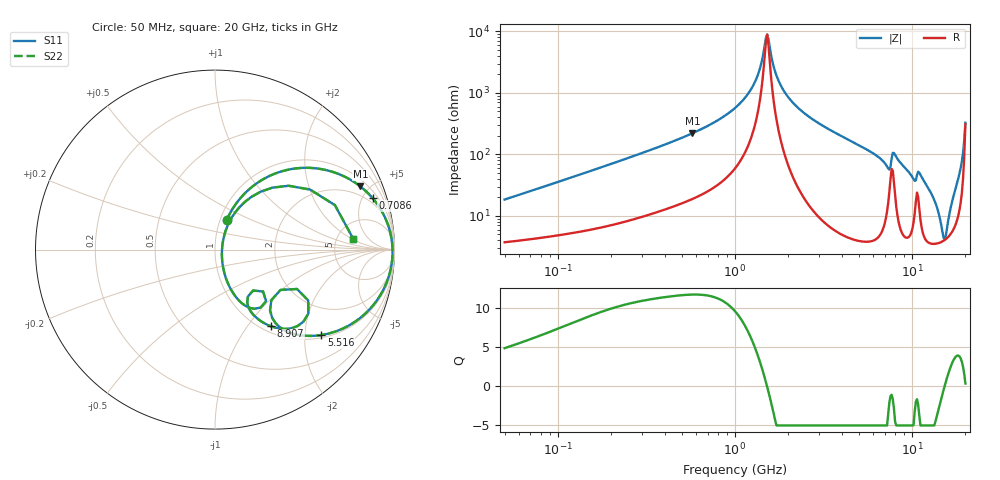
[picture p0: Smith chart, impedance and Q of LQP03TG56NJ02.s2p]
!Murata Part Number: LQP03TG56NJ02
!These Parameters are Measured in Series Mode Connection
!  o--[Z]--o
!Port1  Port2
!  o-------o
!Freq. Start=50[MHz] Stop=20[GHz], 401[Steps]
# Hz S RI R 50
!Freq.(Hz) S11(Real) S11(Imag) S21(Real) S21(Imag) S12(Real) S12(Imag) S22(Real) S22(Imag)
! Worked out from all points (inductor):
!   401 points, 50 MHz to 20 GHz, reference 50 ohm
!   read as one part in series: L = 57 nH near 51.52 MHz
!   highest Q = 11.7 at 574.5 MHz (marker M1), where L = 61 nH
!   self-resonance near 1.498 GHz
!   S11 on the Smith chart (normalised r, x): 50 MHz: 1.07, +0.36; 708.6 MHz: 1.51, +5.89; 5.516 GHz: 1.08, -2.43; 8.907 GHz: 1.10, -1.30; 20 GHz: 7.21, +2.10
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5e7  0.0645 0.1632  0.9355 -0.1632  0.9355 -0.1632  0.0645 0.1632
1.364002e8  0.2147 0.3561  0.7853 -0.3561  0.7853 -0.3561  0.2147 0.3561
3.721004e8  0.6283 0.4408  0.3717 -0.4408  0.3717 -0.4408  0.6283 0.4408
5.745257e8  0.8101 0.3517  0.1899 -0.3517  0.1899 -0.3517  0.8101 0.3517
7.08568e8  0.8776 0.2872  0.1224 -0.2872  0.1224 -0.2872  0.8776 0.2872
1e9  0.9539 0.1638  0.0461 -0.1638  0.0461 -0.1638  0.9539 0.1638
1.289994e9  0.9826 0.0648  0.0174 -0.0648  0.0174 -0.0648  0.9826 0.0648
1.521052e9  0.989 -0.00121  0.011 0.00121  0.011 0.00121  0.989 -0.00121
1.689197e9  0.988 -0.0439  0.012 0.0439  0.012 0.0439  0.988 -0.0439
1.848039e9  0.9839 -0.0809  0.0161 0.0809  0.0161 0.0809  0.9839 -0.0809
2.728004e9  0.9272 -0.2435  0.0728 0.2435  0.0728 0.2435  0.9272 -0.2435
5.515528e9  0.5926 -0.4759  0.4074 0.4759  0.4074 0.4759  0.5926 -0.4759
6.802353e9  0.3962 -0.4539  0.6038 0.4539  0.6038 0.4539  0.3962 -0.4539
7.442007e9  0.3139 -0.2821  0.6861 0.2821  0.6861 0.2821  0.3139 -0.2821
7.901521e9  0.5205 -0.3558  0.4795 0.3558  0.4795 0.3558  0.5205 -0.3558
8.907419e9  0.312 -0.4274  0.688 0.4274  0.688 0.4274  0.312 -0.4274
1.220001e10  0.1102 -0.2557  0.8898 0.2557  0.8898 0.2557  0.1102 -0.2557
1.354865e10  0.0562 -0.1447  0.9438 0.1447  0.9438 0.1447  0.0562 -0.1447
1.527346e10  0.0391 0.000819  0.9609 -0.000819  0.9609 -0.000819  0.0391 0.000819
1.800918e10  0.1649 0.2644  0.8351 -0.2644  0.8351 -0.2644  0.1649 0.2644
1.912117e10  0.4103 0.3556  0.5897 -0.3556  0.5897 -0.3556  0.4103 0.3556
2e10  0.7712 0.0585  0.2288 -0.0585  0.2288 -0.0585  0.7712 0.0585
